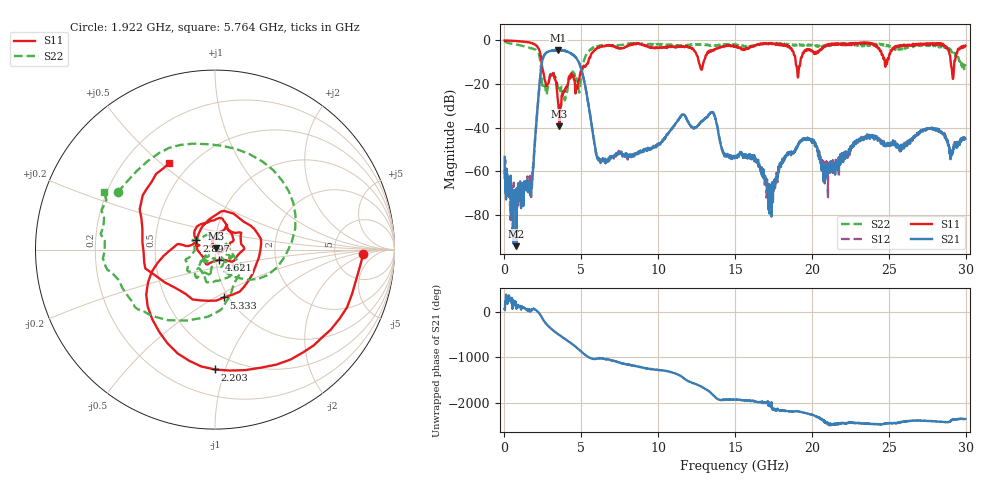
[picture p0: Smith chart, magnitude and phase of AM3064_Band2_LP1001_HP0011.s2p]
# Hz S DB R 50.0
!freq dBS11 angS11 dBS21 angS21 dBS12 angS12 dBS22 angS22
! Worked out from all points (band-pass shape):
!   1600 points, 10 MHz to 29.98 GHz, reference 50 ohm
!   highest |S21| = -4.36 dB at 3.515 GHz (marker M1); lowest = -94.3 dB at 778.5 MHz (marker M2)
!   |S21| within 3 dB of the highest: 2.549 GHz to 4.574 GHz (2.025 GHz wide, 56.9 % of centre)
!   lowest |S11| = -39.4 dB at 3.571 GHz (marker M3), VSWR 1.02, Z = 50.8 + j0.743 ohm
!   |S11| at or under -10 dB: 2.415 GHz to 5.452 GHz (3.037 GHz wide, 77.2 % of centre); 12.64 GHz to 12.95 GHz (311.5 MHz wide, 2.43 % of centre); 18.94 GHz to 19.25 GHz (305.6 MHz wide, 1.6 % of centre)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
!   |S22| runs from -27.5 to -0.2 dB; largest |S21 - S12| = 0.019
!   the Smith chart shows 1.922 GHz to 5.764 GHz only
!   S11 on the Smith chart (normalised r, x): 1.922 GHz: 10, -2; 2.203 GHz: 0.38, -0.92; 2.897 GHz: 0.81, +0.08; 4.621 GHz: 1.04, -0.12; 5.333 GHz: 0.95, -0.55; 5.764 GHz: 0.39, +0.53
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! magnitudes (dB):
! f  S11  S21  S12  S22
! 10 MHz  0.0  -53.4  -59.5  -0.2
! 778.5 MHz  -0.3  -94.3  -70.9  -1.9
! 1.659 GHz  -1.0  -68.1  -62.1  -3.5
! 1.922 GHz  -1.7  -52.4  -52.3  -4.0
! 2.203 GHz  -3.5  -26.5  -26.4  -5.6
! 2.897 GHz  -18.7  -5.0  -5.0  -18.1
! 3.515 GHz  -30.5  -4.4  -4.5  -22.0
! 3.571 GHz  -39.4  -4.4  -4.4  -20.8
! 4.621 GHz  -24.3  -7.6  -7.6  -18.9
! 5.015 GHz  -13.1  -13.7  -13.5  -14.9
! 5.333 GHz  -11.3  -23.9  -23.8  -6.3
! 5.764 GHz  -5.3  -43.2  -43.2  -3.2
! 6.252 GHz  -2.9  -55.6  -56.2  -2.5
! 10 GHz  -3.4  -47.7  -48.0  -1.8
! 13.49 GHz  -4.4  -32.9  -32.7  -2.3
! 15 GHz  -2.6  -53.9  -53.7  -1.9
! 16.34 GHz  -2.4  -54.0  -54.3  -2.3
! 17.33 GHz  -1.3  -76.2  -72.1  -1.5
! 19.99 GHz  -4.6  -46.1  -45.9  -2.0
! 20.91 GHz  -2.1  -59.7  -59.9  -2.4
! 25 GHz  -7.9  -47.7  -47.8  -2.2
! 29.98 GHz  -2.4  -45.1  -46.1  -10.9
